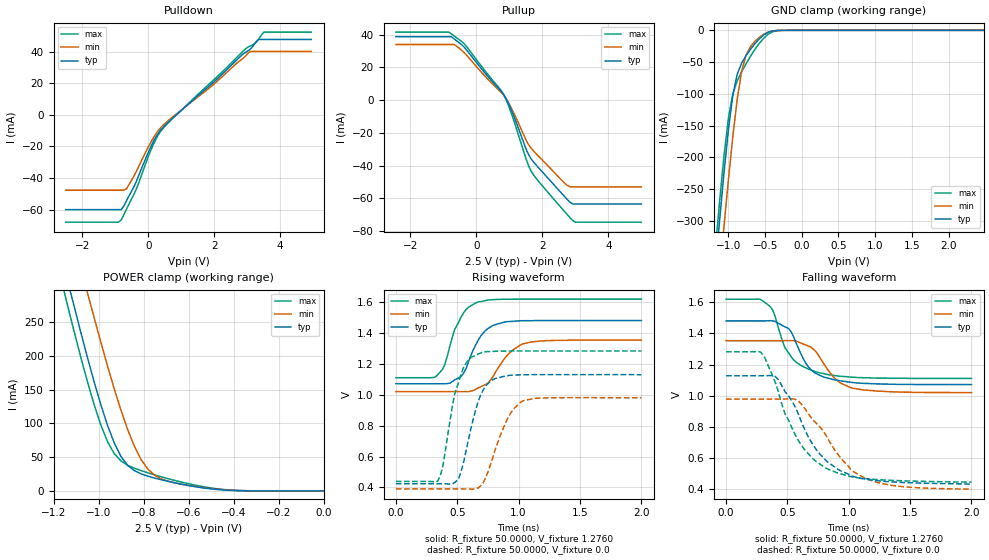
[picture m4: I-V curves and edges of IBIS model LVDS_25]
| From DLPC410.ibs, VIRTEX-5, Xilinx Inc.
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|   Model LVDS_25
[Model]  LVDS_25
Model_type I/O
Polarity   Non-Inverting
Enable   Active-Low
Vinl = 1.025
Vinh = 1.375
Vmeas =  1.2000V
Cref =   0.0F
Rref =   50.0000
Vref =   1.2000V
C_comp   6.0000pF   6.0000pF   6.0000pF
[Model Spec]
Vinl   1.025   0.125   2.025
Vinh   1.375   0.475   2.375
[Temperature Range]   25.0000   85.0000   0.0
[Voltage Range]   2.5000V   2.3750V   2.6250V
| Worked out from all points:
|   slope of the pulldown table from 0 to 0.375 V, typ, clamps not added: 26.5 ohm
|   slope of the pullup table from 0 to 0.375 V, typ, clamps not added: 40.6 ohm
|   GND clamp passes 1 mA (typ) near -0.40 V on its own axis
|   POWER clamp passes 1 mA (typ) near -0.43 V on its own axis
|   rising waveform, R_fixture 50.0000, V_fixture 1.2760: 20-80 % time 150ps typ, 187ps min, 137ps max; typ from 1.07 V to 1.48 V
|   rising waveform, R_fixture 50.0000, V_fixture 0.0: 20-80 % time 134ps typ, 168ps min, 127ps max; typ from 0.424 V to 1.13 V
|   falling waveform, R_fixture 50.0000, V_fixture 1.2760: 20-80 % time 175ps typ, 196ps min, 180ps max; typ from 1.48 V to 1.07 V
|   falling waveform, R_fixture 50.0000, V_fixture 0.0: 20-80 % time 315ps typ, 341ps min, 302ps max; typ from 1.13 V to 0.434 V
[Pulldown]
|Voltage   I(typ)   I(min)   I(max)
-2.5V     -60.03mA   -47.69mA   -67.96mA
-900mV    -60.03mA   -47.69mA   -67.96mA
-820mV    -60.03mA   -47.69mA   -66.53mA
-660mV    -54.45mA   -46.83mA   -59.77mA
-340mV    -41.09mA   -34.91mA   -45.91mA
220mV     -14.44mA   -12.4mA    -15.85mA
380mV     -9.514mA   -8.025mA   -10.28mA
700mV     -2.805mA   -2.01mA    -3.071mA
3.02V     40.46mA    38.93mA    42.87mA
3.34V     47.74mA    40.15mA    47.65mA
3.5V      47.74mA    40.15mA    52.4mA
4.94V     47.74mA    40.15mA    52.4mA
[Pullup]
|Voltage   I(typ)   I(min)   I(max)
-2.44V    38.79mA    34.03mA    41.62mA
-840mV    38.79mA    34.03mA    41.62mA
-680mV    37.57mA    34.03mA    39.33mA
-360mV    32.15mA    28.87mA    34.29mA
840mV     3.045mA    2.654mA    2.897mA
1.08V     -6.986mA   -5.629mA   -9.29mA
1.56V     -32.36mA   -26.5mA    -38.97mA
1.72V     -37.47mA   -30.81mA   -45.35mA
2.68V     -59.05mA   -50.83mA   -68.22mA
2.92V     -63.41mA   -53.01mA   -73.56mA
3V        -63.41mA   -53.01mA   -74.56mA
5V        -63.41mA   -53.01mA   -74.56mA
[GND_clamp]
|Voltage   I(typ)   I(min)   I(max)
-2.5V     -2.205A    -2.201A    -2.217A
-1.18V    -378.2mA   -462.1mA   -347.2mA
-1.12V    -298.9mA   -384.1mA   -268.7mA
-1.06V    -223.8mA   -307.7mA   -197mA
-1V       -156.1mA   -234.6mA   -137.9mA
-940mV    -102.2mA   -166.8mA   -99.83mA
-880mV    -68.83mA   -108.2mA   -79.51mA
-820mV    -51.57mA   -64.34mA   -65.27mA
-700mV    -29.96mA   -25.72mA   -40.91mA
-520mV    -7.399mA   -6.106mA   -12.47mA
-280mV    -46.73uA   -67.7uA    -122.5uA
2.48V     11.1nA     564.1nA    20.99nA
[POWER_clamp]
|Voltage   I(typ)   I(min)   I(max)
-2.49V    2.095A     2.089A     2.108A
-1.17V    354.5mA    443.8mA    318.7mA
-1.14V    315mA      406.5mA    278.4mA
-1.11V    275.8mA    369.1mA    238.4mA
-1.05V    198.7mA    294.6mA    162.8mA
-990mV    128.2mA    220.8mA    97.97mA
-960mV    97.28mA    185.2mA    73.02mA
-900mV    50.94mA    119.4mA    44.35mA
-810mV    25.18mA    45.99mA    30.01mA
-750mV    19mA       23.14mA    23.73mA
-480mV    2.327mA    2.844mA    3.493mA
0V        11.82nA    60.98nA    23.86nA
[Ramp]
dV/dt_r  0.4231/0.1338n   0.3542/0.1682n   0.5065/0.1168n
dV/dt_f  0.1674/85.4286p   0.1368/0.1025n   0.2058/76.3741p
R_load = 50.0000
[Rising Waveform]
R_fixture= 50.0000
V_fixture= 1.2760
V_fixture_min= 1.1870
V_fixture_max= 1.3650
|time   V(typ)   V(min)   V(max)
0s        1.071V     1.02V      1.11V
320ps     1.071V     1.02V      1.114V
400ps     1.071V     1.02V      1.199V
480ps     1.097V     1.02V      1.424V
530ps     1.118V     1.02V      1.502V
670ps     1.352V     1.044V     1.6V
790ps     1.448V     1.116V     1.615V
910ps     1.473V     1.257V     1.618V
1.03ns    1.479V     1.328V     1.619V
2ns       1.48V      1.353V     1.619V
[Rising Waveform]
R_fixture= 50.0000
V_fixture= 0.0
|time   V(typ)   V(min)   V(max)
0s        423.9mV    390mV      438.8mV
340ps     423.8mV    390mV      439.7mV
380ps     424mV      390mV      528.1mV
460ps     423mV      390mV      925.9mV
510ps     455.3mV    390mV      1.078V
610ps     777.2mV    388.8mV    1.241V
750ps     1.072V     500mV      1.279V
910ps     1.123V     846.1mV    1.283V
1.03ns    1.129V     958.8mV    1.283V
2ns       1.129V     980.3mV    1.283V
[Falling Waveform]
R_fixture= 50.0000
V_fixture= 1.2760
V_fixture_min= 1.1870
V_fixture_max= 1.3650
|time   V(typ)   V(min)   V(max)
0s        1.48V      1.353V     1.619V
280ps     1.48V      1.353V     1.618V
360ps     1.481V     1.353V     1.572V
480ps     1.442V     1.354V     1.308V
510ps     1.431V     1.354V     1.275V
650ps     1.209V     1.325V     1.179V
730ps     1.144V     1.285V     1.154V
890ps     1.102V     1.108V     1.129V
1.03ns    1.085V     1.049V     1.119V
2ns       1.072V     1.02V      1.111V
[Falling Waveform]
R_fixture= 50.0000
V_fixture= 0.0
|time   V(typ)   V(min)   V(max)
0s        1.128V     978.5mV    1.282V
280ps     1.128V     978.5mV    1.281V
400ps     1.124V     978.5mV    1.088V
480ps     1.026V     979.2mV    885.7mV
590ps     880.9mV    965.2mV    713.3mV
690ps     709.6mV    863.8mV    611.8mV
810ps     588.7mV    750.7mV    538.1mV
1.01ns    490.6mV    534.9mV    483.2mV
1.13ns    466.3mV    472.5mV    469.4mV
2ns       434.1mV    401.3mV    446.2mV
